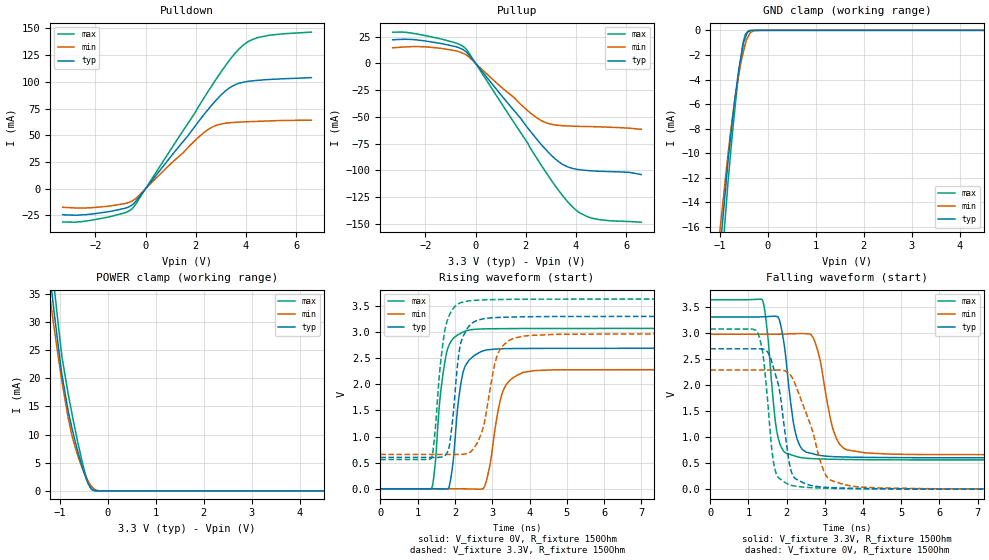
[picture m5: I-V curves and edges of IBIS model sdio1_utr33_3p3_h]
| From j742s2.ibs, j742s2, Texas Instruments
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|   utr33_3p3_h
[Model]   sdio1_utr33_3p3_h
Model_type   I/O
Polarity   Non-Inverting
Enable   Active-High
Vinl = 0
Vinh = 0.8
Vmeas = 1.65
Vref = 3.3
Cref = 2pF
Rref = 100000
|   typ   min   max
C_comp   2.627pF   2.454pF   2.745pF
[Voltage Range]   3.3   2.97   3.63
[Temperature Range]   27   150   -40
[Pullup Reference]   3.3   2.97   3.63
[Pulldown Reference]   0   0   0
[Power Clamp Reference]   3.3   2.97   3.63
[GND Clamp Reference]   0   0   0
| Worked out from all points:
|   slope of the pulldown table from 0 to 0.495 V, typ, clamps not added: 33.3 ohm
|   slope of the pullup table from 0 to 0.495 V, typ, clamps not added: 34 ohm
|   GND clamp passes 1 mA (typ) near -0.51 V on its own axis
|   POWER clamp passes 1 mA (typ) near -0.39 V on its own axis
|   falling waveform, V_fixture 3.3V, R_fixture 150Ohm: 20-80 % time 275ps typ, 362ps min, 233ps max; typ from 3.3 V to 0.6 V
|   rising waveform, V_fixture 0V, R_fixture 150Ohm: 20-80 % time 240ps typ, 328ps min, 249ps max; typ from 0 V to 2.69 V
|   rising waveform, V_fixture 3.3V, R_fixture 150Ohm: 20-80 % time 238ps typ, 379ps min, 247ps max; typ from 0.6 V to 3.3 V
|   falling waveform, V_fixture 0V, R_fixture 150Ohm: 20-80 % time 336ps typ, 598ps min, 233ps max; typ from 2.69 V to 0 V
[Pulldown]
|   Voltage   I(typ)   I(min)   I(max)
-3.3V     -24.38mA   -17.38mA   -31.07mA
-2.023V   -23.32mA   -17.56mA   -28.91mA
-825mV    -18.37mA   -13.92mA   -22.53mA
-557.7mV  -15.53mA   -11.8mA    -19.12mA
-399.3mV  -12.02mA   -9.303mA   -14.67mA
2.363V    70.39mA    53.2mA     86.32mA
2.739V    80.96mA    58.57mA    99.97mA
3.194V    91.69mA    61.27mA    115.5mA
3.749V    98.78mA    62.31mA    131.3mA
4.036V    100.2mA    62.61mA    136.8mA
4.452V    101.4mA    62.98mA    141.3mA
6.6V      103.9mA    64.12mA    146.5mA
[GND Clamp]
|   Voltage   I(typ)   I(min)   I(max)
-3.3V     -160mA     -119.4mA   -217mA
-1.043V   -19.85mA   -17.9mA    -22.95mA
-825mV    -10.42mA   -9.868mA   -12.11mA
-696.3mV  -5.885mA   -5.873mA   -6.719mA
-607.2mV  -3.208mA   -3.606mA   -3.572mA
-528mV    -1.443mA   -2.023mA   -1.27mA
-508.2mV  -1.005mA   -1.707mA   -873.7uA
-468.6mV  -582.9uA   -1.076mA   -329.5uA
-399.3mV  -98.27uA   -434.9uA   -26.03uA
-359.7mV  -27.04uA   -159.3uA   -9.328uA
-171.6mV  -86.92nA   -2.852uA   -107.4nA
6.6V      0A         0A         0A
[Pullup]
|   Voltage   I(typ)   I(min)   I(max)
-3.3V     21.97mA    14.46mA    29.08mA
-2.033V   20.95mA    15.45mA    26.01mA
-518.1mV  13.01mA    9.567mA    16.09mA
-280.5mV  8.28mA     6.239mA    10.26mA
2.046V    -59.48mA   -43.74mA   -73.51mA
2.501V    -72.75mA   -51.94mA   -91.14mA
2.858V    -82.2mA    -56mA      -103.9mA
3.333V    -92.42mA   -58.1mA    -119.7mA
3.877V    -98.38mA   -58.79mA   -134.7mA
4.155V    -99.56mA   -58.98mA   -140mA
4.699V    -100.7mA   -59.26mA   -145.2mA
6.6V      -104mA     -61.73mA   -148.6mA
[POWER Clamp]
|   Voltage   I(typ)   I(min)   I(max)
-3.3V     224.5mA    191.3mA    262.6mA
-1.201V   37.81mA    34.07mA    43.35mA
-1.132V   32.63mA    29.7mA     37.31mA
-1.122V   31.9mA     29.09mA    36.46mA
-953.7mV  20.46mA    19.22mA    23.62mA
-825mV    14.07mA    12.87mA    17.14mA
-686.4mV  9mA        7.916mA    11.1mA
-498.3mV  3.265mA    3.354mA    3.9mA
-399.3mV  1.162mA    1.587mA    1.17mA
-290.4mV  101.1uA    372.4uA    43.55uA
-23.1mV   0A         883.1nA    5.036nA
6.6V      0A         0A         0A
[Ramp]
R_load = 150
|   typ   min   max
dV/dt_r   1.61316/2.39024e-10   1.36857/3.27203e-10   1.84097/2.48096e-10
dV/dt_f   1.61988/2.74389e-10   1.3875/3.61078e-10   1.84245/2.3284e-10
[Falling Waveform]
V_fixture = 3.3V
V_fixture_min = 2.97V
V_fixture_max = 3.63V
R_fixture = 150Ohm
C_fixture = 0F
|   Time   V(typ)   V(min)   V(max)
0s        3.3V       2.969V     3.63V
1.37ns    3.303V     2.97V      3.618V
1.73ns    3.312V     2.97V      1.161V
2ns       2.363V     2.974V     683.8mV
2.185ns   1.239V     2.979V     642.4mV
2.365ns   807.8mV    2.981V     606.2mV
2.745ns   667.7mV    2.814V     583.1mV
3.22ns    623.6mV    1.135V     573mV
3.58ns    615.3mV    752.8mV    568.8mV
10ns      599.9mV    656.8mV    559mV
[Rising Waveform]
V_fixture = 0V
V_fixture_min = 0V
V_fixture_max = 0V
R_fixture = 150Ohm
C_fixture = 0F
|   Time   V(typ)   V(min)   V(max)
0s        356.1uV    920.2uV    207.9uV
1.38ns    186.6uV    605.9uV    10.82mV
1.62ns    -1.908mV   439.9uV    1.853V
1.825ns   6.295mV    473.8uV    2.719V
2.11ns    1.763V     -378uV     2.958V
2.27ns    2.337V     -1.497mV   3.015V
2.795ns   2.647V     41.19mV    3.059V
3.29ns    2.68V      1.873V     3.064V
3.825ns   2.685V     2.225V     3.066V
10ns      2.689V     2.282V     3.068V
[Rising Waveform]
V_fixture = 3.3V
V_fixture_min = 2.97V
V_fixture_max = 3.63V
R_fixture = 150Ohm
C_fixture = 0F
|   Time   V(typ)   V(min)   V(max)
0s        599.9mV    656.8mV    559mV
1.375ns   599.7mV    656.6mV    586.7mV
1.675ns   613.9mV    656.5mV    2.763V
1.845ns   795.6mV    656.5mV    3.311V
2.12ns    2.653V     657.6mV    3.549V
2.36ns    3.096V     681.2mV    3.593V
2.635ns   3.23V      929.6mV    3.609V
3.135ns   3.277V     2.556V     3.621V
3.59ns    3.287V     2.882V     3.625V
10ns      3.3V       2.969V     3.63V
[Falling Waveform]
|Gnd
V_fixture = 0V
V_fixture_min = 0V
V_fixture_max = 0V
R_fixture = 150Ohm
C_fixture = 0F
|   Time   V(typ)   V(min)   V(max)
0s        2.689V     2.282V     3.068V
1.245ns   2.689V     2.282V     2.992V
1.395ns   2.683V     2.282V     2.501V
1.675ns   2.272V     2.282V     437.7mV
1.815ns   1.881V     2.281V     202.4mV
2.045ns   610.4mV    2.232V     93.25mV
2.225ns   201.3mV    2.012V     58.04mV
2.97ns    38.81mV    351.7mV    19.8mV
3.22ns    28.31mV    152.4mV    14.88mV
10ns      353.7uV    920.4uV    207.9uV
